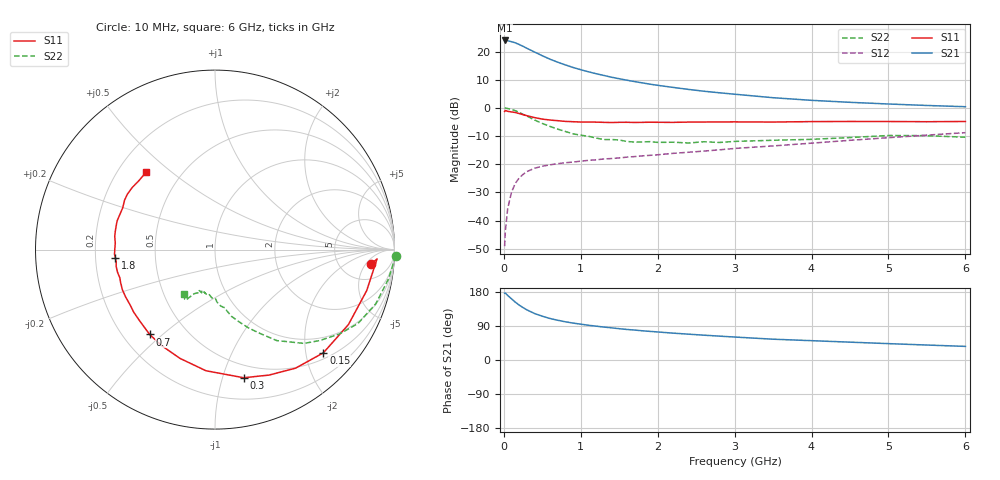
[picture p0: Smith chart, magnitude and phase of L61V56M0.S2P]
!  INFINEON TECHNOLOGIES Small Signal Semiconductors
! BFR380L3 , Si-NPN RF-Transistor in TSLP-3-1
!  Vce=1.5 V,  Ic=6 mA
! Common Emitter S-Parameters:  07. March 2005
#  GHz  S  MA  R  50
! f  S11  S21  S12  S22
! GHz  Mag  Ang  Mag  Ang  Mag  Ang  Mag  Ang
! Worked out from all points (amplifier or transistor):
!   36 points, 10 MHz to 6 GHz, reference 50 ohm
!   highest |S21| = 24.0 dB at 10 MHz (marker M1)
!   |S21| within 3 dB of that: start of sweep to 315.7 MHz
!   unconditionally stable (mu >= 1): 2.326 GHz to 4.83 GHz
!   at 250 MHz: K = 0.19, MSG = 22.8 dB, |S12| = -23.6 dB
!   at 1.4 GHz: K = 0.80, MSG = 14.5 dB, |S12| = -18.0 dB
!   at 6 GHz: K = 0.96, MSG = 4.6 dB, |S12| = -8.7 dB
!   S11 on the Smith chart (normalised r, x): 10 MHz: 10, -7; 150 MHz: 0.63, -2.36; 300 MHz: 0.38, -1.17; 700 MHz: 0.31, -0.45; 1.8 GHz: 0.28, -0.04; 6 GHz: 0.32, +0.41
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0.01  0.8704 -5.4  15.93 176.4  0.0035 86.2  1.01 -2.0
0.02  0.9043 -3.3  15.92 176.5  0.0066 87.2  0.998 -4.0
0.05  0.8756 -15.1  15.74 170.4  0.0163 82.5  0.9809 -9.5
0.1  0.8528 -29.3  15.14 161.3  0.0321 75.8  0.9454 -18.6
0.15  0.8338 -43.6  14.45 152.5  0.046 68.2  0.8968 -27.3
0.2  0.7987 -55.8  13.49 144.8  0.0573 63.3  0.839 -34.0
0.25  0.7612 -66.7  12.53 138.3  0.0661 57.7  0.7735 -40.9
0.3  0.7316 -77.4  11.55 132.2  0.0742 54.4  0.7205 -46.5
0.4  0.6767 -94.3  9.905 122.6  0.0852 48.3  0.613 -55.8
0.5  0.6368 -107.8  8.525 115.5  0.0924 45.2  0.5325 -61.6
0.6  0.6123 -119.0  7.398 109.5  0.0979 43.0  0.4716 -67.1
0.7  0.5966 -127.6  6.543 104.9  0.1025 41.9  0.4226 -71.7
0.9  0.5718 -142.3  5.265 97.4  0.1095 40.9  0.3479 -79.0
1.1  0.5636 -151.9  4.414 91.7  0.1175 41.7  0.3153 -84.4
1.4  0.5531 -163.4  3.536 84.9  0.1266 43.4  0.2762 -90.5
1.8  0.557 -175.3  2.805 77.1  0.1411 46.5  0.2495 -98.4
2.2  0.5567 176.4  2.33 70.9  0.1565 49.3  0.247 -103.1
2.8  0.5669 165.6  1.87 63.0  0.1807 53.2  0.2444 -111.0
3.5  0.5643 155.7  1.528 54.9  0.2122 55.1  0.2675 -114.3
4.5  0.5777 147.6  1.265 47.1  0.267 58.0  0.2989 -118.0
5.5  0.572 137.9  1.112 39.5  0.3302 57.4  0.3232 -121.6
6  0.5773 131.9  1.057 35.9  0.3653 56.2  0.3029 -124.4
